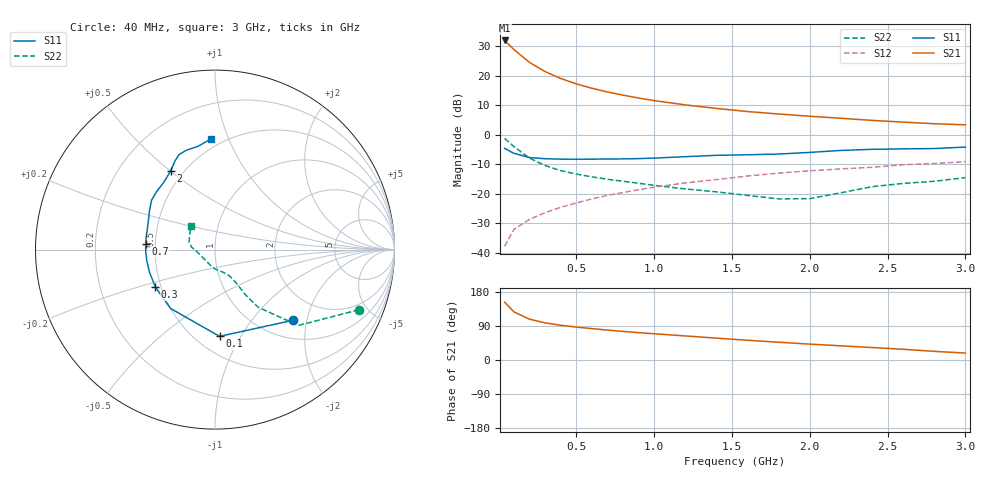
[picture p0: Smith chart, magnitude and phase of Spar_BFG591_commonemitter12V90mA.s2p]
! Filename:  BFG591I.S2P  Version:  4.0
! NXP part #: BFG591  Date: Jun 1994
! Bias condition: Vce=12V; Ic=90mA
#  MHz  S  MA  R  50
! Freq  S11  S21  S12  S22  !GUM [dB]
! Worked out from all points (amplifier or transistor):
!   21 points, 40 MHz to 3 GHz, reference 50 ohm
!   highest |S21| = 31.9 dB at 40 MHz (marker M1)
!   |S21| within 3 dB of that: start of sweep to 98.6 MHz
!   unconditionally stable (mu >= 1): 600.7 MHz to 2.173 GHz
!   at 300 MHz: K = 0.85, MSG = 23.9 dB, |S12| = -26.4 dB
!   at 1 GHz: K = 1.05, MAG = 13.3 dB, |S12| = -17.8 dB
!   at 3 GHz: K = 0.95, MSG = 6.2 dB, |S12| = -9.1 dB
!   S11 on the Smith chart (normalised r, x): 40 MHz: 1.38, -1.66; 100 MHz: 0.65, -0.82; 300 MHz: 0.47, -0.23; 700 MHz: 0.44, +0.03; 2 GHz: 0.43, +0.50; 3 GHz: 0.43, +0.87
40  0.587 -42.1  39.37 152.6  0.013 72.3  0.869 -22.7
100  0.484 -87.0  27.64 127.0  0.025 61.7  0.628 -42.3
200  0.411 -127.1  16.72 107.7  0.037 60.4  0.401 -53.2
300  0.392 -148.1  11.71 98.0  0.048 62.7  0.301 -56.1
400  0.386 -161.3  8.96 91.7  0.059 64.4  0.247 -56.9
500  0.385 -170.7  7.254 86.9  0.07 66.3  0.216 -57.8
600  0.386 -178.2  6.12 82.8  0.082 66.6  0.194 -58.9
700  0.388 175.3  5.294 79.0  0.094 67.1  0.176 -60.3
800  0.39 169.2  4.673 75.5  0.105 67.2  0.163 -62.1
900  0.394 163.2  4.182 72.2  0.117 67.0  0.151 -64.7
1000  0.402 157.8  3.785 69.3  0.129 66.7  0.139 -68.4
1200  0.425 149.1  3.197 63.5  0.153 65.2  0.121 -78.2
1400  0.448 142.1  2.788 57.7  0.174 63.4  0.108 -90.0
1600  0.458 135.5  2.468 52.1  0.2 62.1  0.094 -103.4
1800  0.471 127.4  2.242 46.9  0.224 59.0  0.082 -121.2
2000  0.502 119.5  2.053 41.9  0.245 57.1  0.083 -151.5
2200  0.542 114.3  1.9 37.4  0.264 54.9  0.104 -175.1
2400  0.566 110.7  1.747 32.9  0.281 53.9  0.132 173.8
2600  0.576 106.1  1.635 28.3  0.31 50.2  0.15 163.7
2800  0.583 99.4  1.534 22.8  0.326 46.2  0.163 150.4
3000  0.618 91.9  1.471 18.3  0.349 44.7  0.188 135.2
